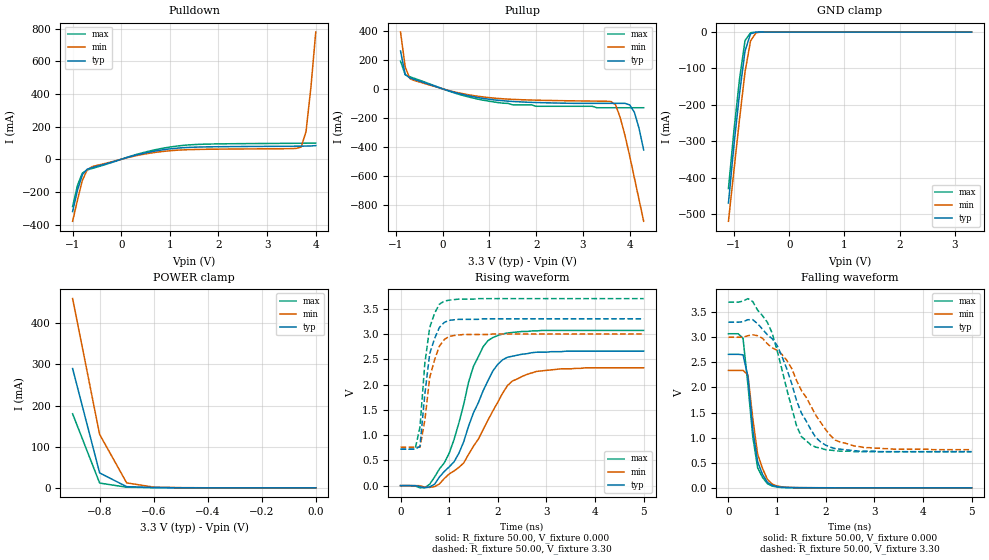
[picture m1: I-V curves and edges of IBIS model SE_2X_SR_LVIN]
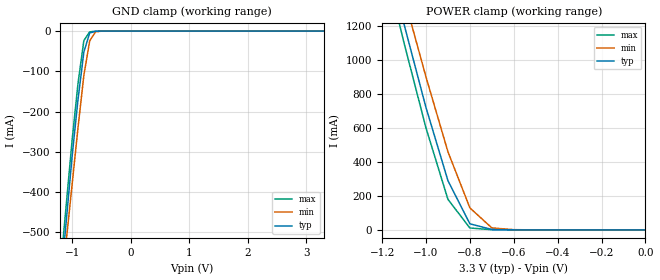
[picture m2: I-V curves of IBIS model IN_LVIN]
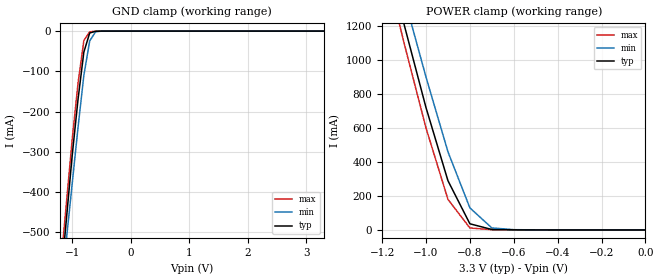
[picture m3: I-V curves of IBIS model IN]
| Integrated Devices Technolgy, Inc
[Ibis Ver]   3.2
[File Name]   9lprs436.ibs
|[File Rev]   1.0 4/28/2009  First release. created by wm
[File Rev]   1.1 3/30/2012
[Date]   3/30/2012
[Source]   Integrated Devices Technolgy, Inc.
[Notes]   Rev 1.0 created by wm
|   Rev 1.1 Updated LPO_R Vmeas lp.
|   Added 9LPRS436C (jitter improvement)
[Disclaimer] Integrated Device Technology, Inc. ("IDT") hereby grants the
   user of this IBIS model a non-exclusive, nontransferable
   license to use this IBIS model under the following terms. The
   user is granted this license only to use the IBIS model and is
   not granted rights to sell, copy (except as needed to run the
   IBIS model), rent, lease or sub-license the IBIS model in
   whole or in part, or in modified form to anyone. The User may
   modify the IBIS model to suit its specific applications, but
   rights to derivative works and such modifications shall belong
   to IDT. This IBIS model is provided on an AS IS" basis and IDT
   makes absolutely no warranty with respect to the information
   contained herein. IDT DISCLAIMS AND CUSTOMER WAIVES ALL
   WARRANTIES, EXPRESS AND IMPLIED, INCLUDING WARRANTIES OF
   MERCHANTABILITY AND FITNESS FOR A PARTICULAR PURPOSE. THE
   ENTIRE RISK AS TO QUALITY AND PERFORMANCE IS WITH THE USER
   ACCORDINGLY, IN NO EVENT SHALL IDT BE LIABLE FOR ANY DIRECT OR
   INDIRECT DAMAGES, WHETHER IN CONTRACT OR TORT, INCLUDING ANY
   LOST PROFITS OR OTHER INCIDENTAL, CONSEQUENTIAL, EXEMPLARY, OR
   PUNITIVE DAMAGES ARISING OUT OF THE USE OR APPLICATION OF THE
   IBIS model. Further, IDT reserves the right to make changes
   without notice to any product herein to improve reliability,
   function, or design. IDT does not convey any license under
   patent rights or any other intellectual property rights,
   including those of third parties. IDT is not obligated to
   provide maintenance or support for the licensed IBIS model.
[Copyright]   Copyright 2006, Integrated Devices Technolgy, Inc. all rights
   reserved
|   COMPONENT: ICS9LPRS436A
[Component]   IDT9LPRS436A
[Manufacturer]   Integrated Device Technology, Inc.
[Package]
| variable   typ   min   max
R_pkg   81.1m   62.2m   100.0m
L_pkg   6.7nH   4.9nH   8.5nH
C_pkg   0.53pF   0.21pF   0.85pF
[Pin]  signal_name   model_name   R_pin   L_pin   C_pin
1   FS3/12_288M_2x   SE_2X_SR_162_IO
2   VDD12_288   POWER
3   PEREQ1#   IN
4   PEREQ2#   IN
5   FS4/PCICLK0_2X   POWER
6   GND   GND
7   VDDPCI   POWER
8   ITP_EN/PCICLK_F0_2x   SE_2X_SR_162_IO
9   PEREQ3#   IN
10   SEL12_4812_48MHz_2x   SE_2X_SR_162_IO
11   VDD   POWER
12   FSA/USB_48MHz_2x   SE_2X_SR_LVIN
13   GND   GND
14   DOTT_96MHzLR   LPO_R
15   DOTC_96MHzLR   LPO_R
16   FSB   IN_LVIN
17   GNDSATA   GND
18   SATAT_LR/PCIeT_LR3   LPO_R
19   SATAC_LR/PCIeC_LR3   LPO_R
20   VDDSATA   POWER
21   PCIeT_LR0   LPO_R
22   PCIeC_LR0   LPO_R
23   PCIeT_LR1   LPO_R
24   PCIeC_LR1   LPO_R
25   GND   GND
26   VDDPCIEX   POWER
27   CPUITPT_LR2PCIeT_LR2   LPO_R
28   CPUITPC_LR2PCIeC_LR2   LPO_R
29   CPUC_LR1   LPO_R
30   CPUT_LR1   LPO_R
31   VDDCPU   POWER
32   CPUC_LR1   LPO_R
33   CPUT_LR1   LPO_R
34   GND   GND
35   SCLK   SCL
36   SDATA   SDA
37   CPU_STOP#   IN
38   PCI&PCIEX_STOP#   IN
39   X2_25   XTL_OUT
40   X1_25   XT1
41   GND   GND
42   25M   SE_1X
43   VDDSUSP   POWER
44   Vtt_PwrGd/WOL_STOP#   IN
45   VDDREF   POWER
46   REF0/FSLC   SE_2X_SR_LVIN
47   GND   GND
48   GND   GND
[Diff Pin]   inv_pin   vdiff   tdelay_typ   tdelay_min   tdelay_max
14   15   NA   NA
18   19   NA   NA
21   22   NA   NA
23   24   NA   NA
28   27   NA   NA
30   29   NA   NA
33   32   NA   NA
|   COMPONENT: ICS9LPRS436C
[Component]   IDT9LPRS436C
[Manufacturer]   Integrated Device Technology, Inc.
[Package]
| variable   typ   min   max
R_pkg   81.1m   62.2m   100.0m
L_pkg   6.7nH   4.9nH   8.5nH
C_pkg   0.53pF   0.21pF   0.85pF
[Pin]  signal_name   model_name   R_pin   L_pin   C_pin
1   FS3/12_288M_2x   SE_2X_SR_162_IO
2   VDD12_288   POWER
3   PEREQ1#   IN
4   PEREQ2#   IN
5   FS4/PCICLK0_2X   POWER
6   GND   GND
7   VDDPCI   POWER
8   ITP_EN/PCICLK_F0_2x   SE_2X_SR_162_IO
9   PEREQ3#   IN
10   SEL12_4812_48MHz_2x   SE_2X_SR_162_IO
11   VDD   POWER
12   FSA/USB_48MHz_2x   SE_2X_SR_LVIN
13   GND   GND
14   DOTT_96MHzLR   LPO_R
15   DOTC_96MHzLR   LPO_R
16   FSB   IN_LVIN
17   GNDSATA   GND
18   SATAT_LR/PCIeT_LR3   LPO_R
19   SATAC_LR/PCIeC_LR3   LPO_R
20   VDDSATA   POWER
21   PCIeT_LR0   LPO_R
22   PCIeC_LR0   LPO_R
23   PCIeT_LR1   LPO_R
24   PCIeC_LR1   LPO_R
25   GND   GND
26   VDDPCIEX   POWER
27   CPUITPT_LR2PCIeT_LR2   LPO_R
28   CPUITPC_LR2PCIeC_LR2   LPO_R
29   CPUC_LR1   LPO_R
30   CPUT_LR1   LPO_R
31   VDDCPU   POWER
32   CPUC_LR1   LPO_R
33   CPUT_LR1   LPO_R
34   GND   GND
35   SCLK   SCL
36   SDATA   SDA
37   CPU_STOP#   IN
38   PCI&PCIEX_STOP#   IN
39   X2_25   XTL_OUT
40   X1_25   XT1
41   GND   GND
42   25M   SE_1X
43   VDDSUSP   POWER
44   Vtt_PwrGd/WOL_STOP#   IN
45   VDDREF   POWER
46   REF0/FSLC   SE_2X_SR_LVIN
47   GND   GND
48   GND   GND
[Diff Pin]   inv_pin   vdiff   tdelay_typ   tdelay_min   tdelay_max
14   15   NA   NA
18   19   NA   NA
21   22   NA   NA
23   24   NA   NA
28   27   NA   NA
30   29   NA   NA
33   32   NA   NA
| Models and submodels in the file (10): SE_2X_SR_LVIN (I/O), IN_LVIN (Input), IN (Input), SE_2X_SR_162_IO (I/O), SDA (I/O_open_drain), SCL (Input), LPO_R (Output), XT1 (Input), XTL_OUT (Output), SE_1X (Output)
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|   Model SE_2X_SR_LVIN
[Model]   SE_2X_SR_LVIN
Model_type   I/O
Polarity   Inverting
Vinl =   0.35V
Vinh =   0.7V
Vmeas =   1.50V
Cref =   5.00pF
Rref =  0.000
Vref =   1.50V
C_comp   3.40pF   2.85pF   3.95pF
[Temperature Range]   27.00   70.00   0.000
[Voltage Range]   3.30V   3.00V   3.70V
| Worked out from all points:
|   slope of the pulldown table from 0 to 0.495 V, typ, clamps not added: 12.7 ohm
|   slope of the pullup table from 0 to 0.495 V, typ, clamps not added: 11.3 ohm
|   GND clamp passes 1 mA (typ) near -0.61 V on its own axis
|   POWER clamp passes 1 mA (typ) near -0.61 V on its own axis
|   rising waveform, R_fixture 50.00, V_fixture 0.000: 20-80 % time 689ps typ, 813ps min, 564ps max; typ from 0 V to 2.66 V
|   rising waveform, R_fixture 50.00, V_fixture 3.30: 20-80 % time 214ps typ, 238ps min, 184ps max; typ from 0.72 V to 3.3 V
|   falling waveform, R_fixture 50.00, V_fixture 0.000: 20-80 % time 189ps typ, 228ps min, 209ps max; typ from 2.66 V to 0 V
|   falling waveform, R_fixture 50.00, V_fixture 3.30: 20-80 % time 627ps typ, 776ps min, 490ps max; typ from 3.3 V to 0.72 V
[Pulldown]
| voltage   I(typ)   I(min)   I(max)
|  -3.30   -4.15A   -4.00A   -4.25A
|  -3.10   -3.81A   -3.68A   -3.90A
|  -2.90   -3.47A   -3.36A   -3.55A
|  -2.70   -3.13A   -3.04A   -3.19A
|  -2.50   -2.79A   -2.72A   -2.84A
|  -2.30   -2.46A   -2.40A   -2.49A
|  -2.10   -2.12A   -2.08A   -2.14A
|  -1.90   -1.78A   -1.77A   -1.79A
|  -1.70   -1.45A   -1.45A   -1.45A
|  -1.50   -1.12A   -1.14A   -1.10A
-1V       -320mA     -380mA     -290mA
-900mV    -190mA     -250mA     -160mA
-800mV    -94.69mA   -130mA     -84.74mA
-700mV    -60.71mA   -64.73mA   -65.52mA
-600mV    -51.06mA   -45.2mA    -56.5mA
400mV     32.6mA     27.52mA    37.03mA
1.2V      69.5mA     56.57mA    82.87mA
3.5V      80.08mA    65.45mA    97.87mA
3.7V      80.56mA    75.12mA    98.32mA
3.8V      80.96mA    170mA      98.58mA
3.9V      81.72mA    440mA      98.88mA
4V        83.73mA    780mA      99.22mA
|   4.10   0.11A   1.16A   99.62mA
|   4.20   0.31A   1.55A   0.10A
|   4.30   0.66A   1.95A   0.10A
|   4.50   1.46A   2.77A   0.11A
|   4.70   2.32A   3.59A   0.58A
|   4.90   3.19A   4.43A   1.41A
|   5.10   4.07A   5.27A   2.30A
|   5.30   4.96A   6.11A   3.20A
|   5.50   5.85A   6.96A   4.12A
|   5.70   6.75A   7.81A   5.04A
|   5.90   7.64A   8.66A   5.97A
|   6.10   8.54A   9.51A   6.89A
|   6.60   10.80A   11.65A   9.23A
[Pullup]
| voltage   I(typ)   I(min)   I(max)
|  -3.30   10.68A   10.27A   10.94A
|  -3.10   9.78A   9.42A   10.01A
|  -2.90   8.88A   8.57A   9.08A
|  -2.70   7.99A   7.73A   8.16A
|  -2.50   7.09A   6.88A   7.23A
|  -2.30   6.20A   6.04A   6.30A
|  -2.10   5.31A   5.20A   5.38A
|  -1.90   4.42A   4.36A   4.46A
|  -1.70   3.54A   3.53A   3.55A
|  -1.50   2.67A   2.70A   2.64A
|  -1.00   0.59A   0.73A   0.50A
-900mV    260mA      390mA      190mA
-800mV    98.09mA    150mA      96.73mA
-700mV    74.34mA    69.92mA    82.79mA
-600mV    63.81mA    56.49mA    71.52mA
500mV     -44.25mA   -37.82mA   -51.47mA
1.5V      -86.95mA   -72.42mA   -110mA
3.5V      -100mA     -85.41mA   -130mA
3.7V      -100mA     -110mA     -130mA
3.9V      -100mA     -320mA     -130mA
4.1V      -160mA     -610mA     -130mA
4.2V      -270mA     -760mA     -130mA
4.3V      -420mA     -910mA     -130mA
|   4.50   -0.73A   -1.22A   -0.15A
|   4.70   -1.06A   -1.54A   -0.40A
|   4.90   -1.39A   -1.85A   -0.72A
|   5.10   -1.72A   -2.17A   -1.06A
|   5.30   -2.06A   -2.49A   -1.40A
|   5.50   -2.39A   -2.81A   -1.75A
|   5.70   -2.73A   -3.13A   -2.10A
|   5.90   -3.07A   -3.45A   -2.45A
|   6.10   -3.41A   -3.77A   -2.80A
|   6.60   -4.26A   -4.58A   -3.68A
[GND_clamp]
| voltage   I(typ)   I(min)   I(max)
|  -3.30   -4.15A   -4.00A   -4.25A
|  -3.20   -3.98A   -3.84A   -4.07A
|  -3.10   -3.81A   -3.68A   -3.90A
|  -3.00   -3.64A   -3.52A   -3.72A
|  -2.90   -3.47A   -3.36A   -3.55A
|  -2.80   -3.30A   -3.20A   -3.37A
|  -2.70   -3.13A   -3.04A   -3.19A
|  -2.60   -2.96A   -2.88A   -3.02A
|  -2.50   -2.79A   -2.72A   -2.84A
|  -2.40   -2.62A   -2.56A   -2.67A
|  -2.30   -2.45A   -2.40A   -2.49A
|  -2.20   -2.29A   -2.24A   -2.32A
|  -2.10   -2.12A   -2.08A   -2.14A
|  -2.00   -1.95A   -1.92A   -1.97A
|  -1.90   -1.78A   -1.76A   -1.79A
|  -1.80   -1.61A   -1.61A   -1.62A
|  -1.70   -1.45A   -1.45A   -1.45A
|  -1.60   -1.28A   -1.29A   -1.27A
|  -1.50   -1.12A   -1.14A   -1.10A
|  -1.40   -0.95A   -0.98A   -0.93A
|  -1.30   -0.79A   -0.83A   -0.76A
|  -1.20   -0.63A   -0.67A   -0.59A
-1.1V     -470mA     -520mA     -430mA
-1V       -310mA     -380mA     -270mA
-900mV    -170mA     -240mA     -130mA
-800mV    -52.1mA    -110mA     -23.59mA
-700mV    -4.69mA    -24.29mA   -1.84mA
-600mV    -430uA     -1.9mA     -210uA
-400mV    -1.76uA    -10.19uA   -470nA
3.3V      150pA      24.14uA    -330pA
[POWER_clamp]
| voltage   I(typ)   I(min)   I(max)
|  -3.30   13.34A   12.83A   13.67A
|  -3.20   12.78A   12.30A   13.09A
|  -3.10   12.22A   11.77A   12.51A
|  -3.00   11.66A   11.24A   11.93A
|  -2.90   11.10A   10.71A   11.35A
|  -2.80   10.54A   10.18A   10.77A
|  -2.70   9.98A   9.66A   10.19A
|  -2.60   9.42A   9.13A   9.61A
|  -2.50   8.86A   8.60A   9.03A
|  -2.40   8.31A   8.07A   8.46A
|  -2.30   7.75A   7.54A   7.88A
|  -2.20   7.19A   7.02A   7.30A
|  -2.10   6.64A   6.49A   6.73A
|  -2.00   6.08A   5.97A   6.15A
|  -1.90   5.53A   5.45A   5.58A
|  -1.80   4.97A   4.92A   5.00A
|  -1.70   4.42A   4.40A   4.43A
|  -1.60   3.88A   3.89A   3.86A
|  -1.50   3.33A   3.37A   3.30A
|  -1.40   2.79A   2.86A   2.74A
|  -1.30   2.25A   2.35A   2.18A
|  -1.20   1.72A   1.85A   1.63A
|  -1.10   1.21A   1.37A   1.10A
|  -1.00   0.72A   0.90A   0.60A
-900mV    290mA      460mA      180mA
-800mV    36.29mA    130mA      11.65mA
-700mV    2.83mA     12.05mA    1.52mA
-600mV    760uA      1.75mA     430uA
-500mV    190uA      510uA      90.12uA
-400mV    36.78uA    130uA      14.36uA
-300mV    5.51uA     24.14uA    1.75uA
-200mV    600nA      3.69uA     140nA
-100mV    40.72nA    380nA      6.97nA
0V        150pA      200pA      160pA
[Ramp]
| variable   typ   min   max
dV/dt_r   1.60/0.68n   1.40/0.84n   1.84/0.57n
dV/dt_f   1.55/0.62n   1.34/0.77n   1.79/0.50n
R_load = 50.00
[Rising Waveform]
R_fixture = 50.00
V_fixture = 0.000
V_fixture_min = 0.000
V_fixture_max = 0.000
| time   V(typ)   V(min)   V(max)
0s        0V         1.34uV     0V
500ps     -41.76mV   -33.07mV   -39.36mV
700ps     28.97mV    -20.58mV   170mV
900ps     280mV      140mV      450mV
1.2ns     640mV      360mV      1.24V
1.5ns     1.44V      780mV      2.36V
1.8ns     2.08V      1.3V       2.87V
2.2ns     2.54V      1.98V      3.02V
2.6ns     2.61V      2.2V       3.05V
5ns       2.66V      2.33V      3.07V
[Rising Waveform]
R_fixture = 50.00
V_fixture = 3.30
V_fixture_min = 3.00
V_fixture_max = 3.70
| time   V(typ)   V(min)   V(max)
0s        720mV      760mV      720mV
300ps     720mV      760mV      720mV
400ps     780mV      760mV      1.16V
500ps     1.81V      1.29V      2.42V
600ps     2.61V      2.14V      3.13V
700ps     2.91V      2.49V      3.41V
800ps     3.13V      2.76V      3.59V
900ps     3.23V      2.89V      3.65V
1.3ns     3.29V      2.99V      3.69V
5ns       3.3V       3V         3.7V
[Falling Waveform]
R_fixture = 50.00
V_fixture = 0.000
V_fixture_min = 0.000
V_fixture_max = 0.000
| time   V(typ)   V(min)   V(max)
0s        2.66V      2.34V      3.07V
200ps     2.66V      2.34V      3.07V
300ps     2.65V      2.34V      2.98V
400ps     2.22V      2.25V      2.06V
500ps     1.16V      1.39V      1.02V
600ps     520mV      670mV      400mV
800ps     110mV      170mV      83.3mV
1ns       24.56mV    35.51mV    15.19mV
1.3ns     4.76mV     7.41mV     3.26mV
5ns       1.01uV     4.93uV     0V
[Falling Waveform]
R_fixture = 50.00
V_fixture = 3.30
V_fixture_min = 3.00
V_fixture_max = 3.70
| time   V(typ)   V(min)   V(max)
0s        3.3V       3V         3.7V
400ps     3.35V      3.03V      3.77V
800ps     3.05V      2.87V      3.3V
1ns       2.84V      2.74V      2.74V
1.2ns     2.37V      2.54V      1.96V
1.4ns     1.74V      2.14V      1.24V
1.7ns     1.15V      1.62V      850mV
2.2ns     780mV      950mV      740mV
2.6ns     740mV      830mV      720mV
5ns       720mV      760mV      720mV
|   Model IN_LVIN
[Model]   IN_LVIN
Model_type   Input
Polarity   Inverting
Vinl =   0.35V
Vinh =   0.7V
C_comp   3.40pF   2.85pF   3.95pF
[Temperature Range]   27.00   70.00   0.000
[Voltage Range]   3.30V   3.00V   3.70V
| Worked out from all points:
|   GND clamp passes 1 mA (typ) near -0.61 V on its own axis
|   POWER clamp passes 1 mA (typ) near -0.61 V on its own axis
[GND_clamp]
| voltage   I(typ)   I(min)   I(max)
-3.3V     -4.15A     -4A        -4.25A
-1.2V     -630mA     -670mA     -590mA
-1.1V     -470mA     -520mA     -430mA
-1V       -310mA     -380mA     -270mA
-900mV    -170mA     -240mA     -130mA
-800mV    -52.1mA    -110mA     -23.59mA
-700mV    -4.69mA    -24.29mA   -1.84mA
-600mV    -430uA     -1.9mA     -210uA
-500mV    -36.26uA   -150uA     -14.73uA
3.3V      150pA      24.14uA    -330pA
[POWER_clamp]
| voltage   I(typ)   I(min)   I(max)
-3.3V     13.34A     12.83A     13.67A
-1.2V     1.72A      1.85A      1.63A
-1.1V     1.21A      1.37A      1.1A
-1V       720mA      900mA      600mA
-900mV    290mA      460mA      180mA
-800mV    36.29mA    130mA      11.65mA
-700mV    2.83mA     12.05mA    1.52mA
-600mV    760uA      1.75mA     430uA
0V        150pA      200pA      160pA
|   Model IN
[Model]   IN
Model_type   Input
Polarity   Inverting
Vinl =   0.80V
Vinh =   2.00V
C_comp   3.40pF   2.85pF   3.95pF
[Temperature Range]   27.00   70.00   0.000
[Voltage Range]   3.30V   3.00V   3.70V
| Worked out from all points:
|   GND clamp passes 1 mA (typ) near -0.61 V on its own axis
|   POWER clamp passes 1 mA (typ) near -0.61 V on its own axis
[GND_clamp]
| voltage   I(typ)   I(min)   I(max)
-3.3V     -4.16A     -4.01A     -4.26A
-1.2V     -630mA     -670mA     -590mA
-1.1V     -470mA     -520mA     -430mA
-1V       -310mA     -380mA     -270mA
-900mV    -170mA     -240mA     -130mA
-800mV    -52.15mA   -110mA     -23.62mA
-700mV    -4.69mA    -24.32mA   -1.84mA
-600mV    -430uA     -1.9mA     -210uA
-500mV    -36.28uA   -150uA     -14.74uA
3.3V      150pA      24.16uA    -320pA
[POWER_clamp]
| voltage   I(typ)   I(min)   I(max)
-3.3V     13.35A     12.84A     13.68A
-1.2V     1.72A      1.85A      1.63A
-1.1V     1.21A      1.37A      1.1A
-1V       720mA      900mA      600mA
-900mV    290mA      460mA      180mA
-800mV    36.36mA    130mA      11.68mA
-700mV    2.84mA     12.08mA    1.52mA
-600mV    760uA      1.75mA     430uA
0V        150pA      200pA      170pA
